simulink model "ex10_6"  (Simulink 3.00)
settings: Solver=ode45  SolverMode=SingleTasking  StartTime=0.0  StopTime=10.0  FixedStep=0.1  RelTol=1e-3  AbsTol=1e-6

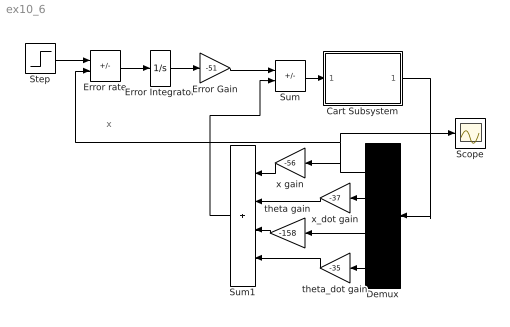
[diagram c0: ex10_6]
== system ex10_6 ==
  note: x
  Cart Subsystem : Subsystem  mask{M=2, m=.1, l=.5}
      mask prompts: M "Cart mass:"; m "Pendulum mass:"; l "Pendulum lenght:"
  Demux : Demux  Orientation=left  Outputs=4
  Error Gain : Gain  Gain=-51  SaturateOnIntegerOverflow=on
  Error Integrator : Integrator  ExternalReset=none  InitialConditionSource=internal  InitialCondition=0  LimitOutput=off  UpperSaturationLimit=2  LowerSaturationLimit=-2  ShowSaturationPort=off  ShowStatePort=off  AbsoluteTolerance=auto
  Error rate : Sum  Inputs=+-  SaturateOnIntegerOverflow=on
  Scope : Scope
  Step : Step  Time=1  Before=0  After=1  SampleTime=-1
  Sum : Sum  Inputs=+-  SaturateOnIntegerOverflow=on
  Sum1 : Sum  Orientation=left  Inputs=++++  SaturateOnIntegerOverflow=on
  theta gain : Gain  Orientation=left  Gain=-158  SaturateOnIntegerOverflow=on
  theta_dot gain : Gain  Orientation=left  Gain=-35  SaturateOnIntegerOverflow=on
  x gain : Gain  Orientation=left  Gain=-56  SaturateOnIntegerOverflow=on
  x_dot gain : Gain  Orientation=left  Gain=-37  SaturateOnIntegerOverflow=on
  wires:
  Error rate/1 -> Error Integrator/1
  Cart Subsystem/1(Out1) -> Demux/1
  Demux/1 -> Scope/1, Error rate/2, x gain/1
  Sum1/1 -> Sum/2
  x gain/1 -> Sum1/1
  x_dot gain/1 -> Sum1/2
  theta gain/1 -> Sum1/3
  theta_dot gain/1 -> Sum1/4
  Demux/4 -> theta_dot gain/1
  Demux/3 -> theta gain/1
  Demux/2 -> x_dot gain/1
  Step/1 -> Error rate/1
  Error Integrator/1 -> Error Gain/1
  Error Gain/1 -> Sum/1
  Sum/1 -> Cart Subsystem/1(In1)

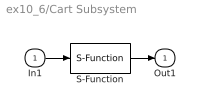
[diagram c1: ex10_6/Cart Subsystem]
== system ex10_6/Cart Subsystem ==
  In1 : Inport  Port=1  PortWidth=-1  SampleTime=-1  DataType=auto
  S-Function : S-Function  FunctionName=s_xmp2  Parameters=M,m,l  PortCounts=[]  SFunctionModules=''
  Out1 : Outport  Port=1  InitialOutput=0
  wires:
  In1/1 -> S-Function/1
  S-Function/1 -> Out1/1
